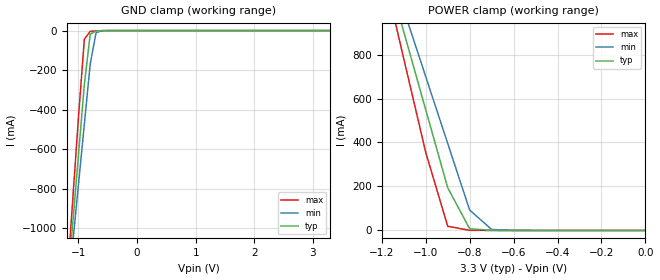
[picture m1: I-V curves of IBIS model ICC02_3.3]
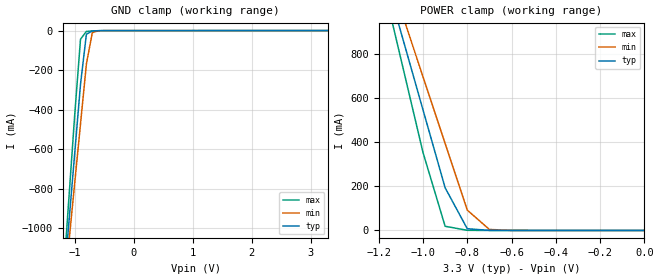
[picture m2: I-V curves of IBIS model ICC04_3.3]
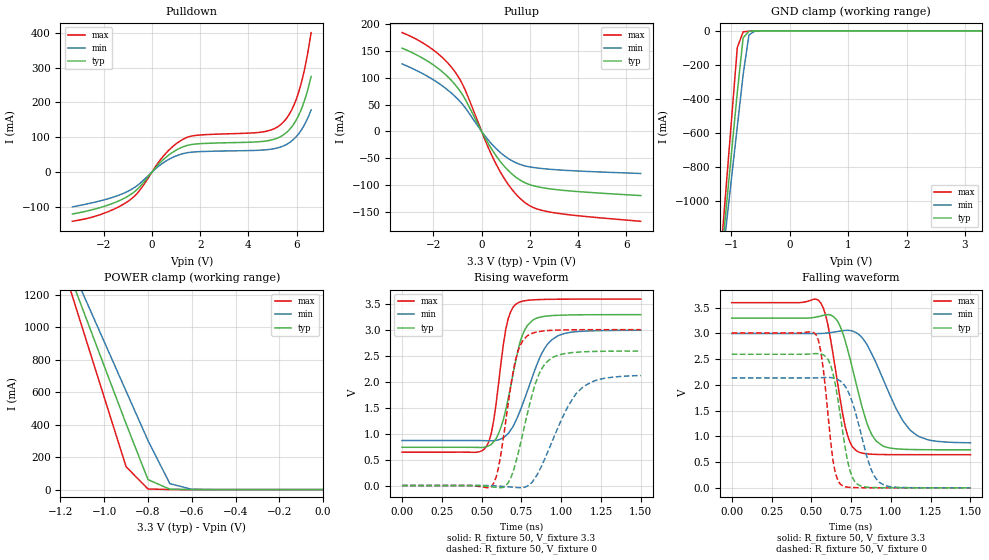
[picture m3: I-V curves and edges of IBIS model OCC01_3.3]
|   MPC9350   I B I S   M O D E L   |
|   F R E E S C A L E   S E M I C O N D U C T O R   |
[IBIS Ver]   3.2
[File name]   mpc9350.ibs
[File Rev]   1.0
[Date]   01-Apr-05 10:30:01 AM
[Source]   This file was generated from transistor-level
|   simulations
[Notes]   This file contains data for 3.3V and 2.5 V
|   applications.
[Disclaimer]   This information is for modeling purposes only,
|   and is not guaranteed.
[Copyright]   Copyright 2005, Freescale Semiconductor.,
|   All Rights Reserved.
|   MPC9350
|   --- 3.3V Application ---
|   C O M P O N E N T  D E S C R I P T I O N
[Component]   mpc9350_3.3v
[Manufacturer]   Freescale Semiconductor
[Package]
R_pkg   40m   40m   40m
L_pkg   0.5nH   0.5nH   0.5nH
C_pkg   0.23pF   0.23pF   0.23pF
[Pin] signal_name   model_name   R_pin   L_pin   C_pin
1   VCCA   POWER   40m   0.5nH   0.23pF
2   FBSEL   ICC04_3.3   40m   0.5nH   0.23pF
3   FSELA   ICC04_3.3   40m   0.5nH   0.23pF
4   FSELB   ICC04_3.3   40m   0.5nH   0.23pF
5   FSELC   ICC04_3.3   40m   0.5nH   0.23pF
6   FSELD   ICC04_3.3   40m   0.5nH   0.23pF
7   GND   GND   40m   0.5nH   0.23pF
|8   XTAL1   NA   40m   0.5nH   0.23pF
|9   XTAL2   NA   40m   0.5nH   0.23pF
10   OEB   ICC04_3.3   40m   0.5nH   0.23pF
11   VCCO   POWER   40m   0.5nH   0.23pF
12   QD4   OCC01_3.3   40m   0.5nH   0.23pF
13   GND   GND   40m   0.5nH   0.23pF
14   QD3   OCC01_3.3   40m   0.5nH   0.23pF
15   VCCO   POWER   40m   0.5nH   0.23pF
16   QD2   OCC01_3.3   40m   0.5nH   0.23pF
17   GND   GND   40m   0.5nH   0.23pF
18   QD1   OCC01_3.3   40m   0.5nH   0.23pF
19   VCCO   POWER   40m   0.5nH   0.23pF
20   QD0   OCC01_3.3   40m   0.5nH   0.23pF
21   GND   GND   40m   0.5nH   0.23pF
22   QC1   OCC01_3.3   40m   0.5nH   0.23pF
23   VCCO   POWER   40m   0.5nH   0.23pF
24   QC0   OCC01_3.3   40m   0.5nH   0.23pF
25   GND   GND   40m   0.5nH   0.23pF
26   QB   OCC01_3.3   40m   0.5nH   0.23pF
27   VCCO   POWER   40m   0.5nH   0.23pF
28   QA   OCC01_3.3   40m   0.5nH   0.23pF
29   GND   GND   40m   0.5nH   0.23pF
30   TCLK   ICC04_3.3   40m   0.5nH   0.23pF
31   PLL_EN   ICC02_3.3   40m   0.5nH   0.23pF
32   REF_SEL   ICC04_3.3   40m   0.5nH   0.23pF
|[Diff Pin] inv_pin vdiff   tdelay_typ tdelay_min tdelay_max
|8   9   0.0   0.0   0.0   0.0
|   MPC9350
|   --- 2.5V Application ----
|   C O M P O N E N T  D E S C R I P T I O N
[Component]   mpc9350_2.5v
[Manufacturer]   Freescale Semiconductor
[Package]
R_pkg   40m   40m   40m
L_pkg   0.5nH   0.5nH   0.5nH
C_pkg   0.23pF   0.23pF   0.23pF
[Pin] signal_name   model_name   R_pin   L_pin   C_pin
1   VCCA   POWER   40m   0.5nH   0.23pF
2   FBSEL   ICC04_2.5   40m   0.5nH   0.23pF
3   FSELA   ICC04_2.5   40m   0.5nH   0.23pF
4   FSELB   ICC04_2.5   40m   0.5nH   0.23pF
5   FSELC   ICC04_2.5   40m   0.5nH   0.23pF
6   FSELD   ICC04_2.5   40m   0.5nH   0.23pF
7   GND   GND   40m   0.5nH   0.23pF
|8   XTAL1   NA   40m   0.5nH   0.23pF
|9   XTAL2   NA   40m   0.5nH   0.23pF
10   OEB   ICC04_2.5   40m   0.5nH   0.23pF
11   VCCO   POWER   40m   0.5nH   0.23pF
12   QD4   OCC01_2.5   40m   0.5nH   0.23pF
13   GND   GND   40m   0.5nH   0.23pF
14   QD3   OCC01_2.5   40m   0.5nH   0.23pF
15   VCCO   POWER   40m   0.5nH   0.23pF
16   QD2   OCC01_2.5   40m   0.5nH   0.23pF
17   GND   GND   40m   0.5nH   0.23pF
18   QD1   OCC01_2.5   40m   0.5nH   0.23pF
19   VCCO   POWER   40m   0.5nH   0.23pF
20   QD0   OCC01_2.5   40m   0.5nH   0.23pF
21   GND   GND   40m   0.5nH   0.23pF
22   QC1   OCC01_2.5   40m   0.5nH   0.23pF
23   VCCO   POWER   40m   0.5nH   0.23pF
24   QC0   OCC01_2.5   40m   0.5nH   0.23pF
25   GND   GND   40m   0.5nH   0.23pF
26   QB   OCC01_2.5   40m   0.5nH   0.23pF
27   VCCO   POWER   40m   0.5nH   0.23pF
28   QA   OCC01_2.5   40m   0.5nH   0.23pF
29   GND   GND   40m   0.5nH   0.23pF
30   TCLK   ICC04_2.5   40m   0.5nH   0.23pF
31   PLL_EN   ICC02_2.5   40m   0.5nH   0.23pF
32   REF_SEL   ICC04_2.5   40m   0.5nH   0.23pF
| Models and submodels in the file (6): ICC02_3.3 (Input), ICC04_3.3 (Input), OCC01_3.3 (3-state), ICC02_2.5 (Input), ICC04_2.5 (Input), OCC01_2.5 (3-state)
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|[Diff Pin] inv_pin vdiff   tdelay_typ tdelay_min tdelay_max
|8   9   0.0   0.0   0.0   0.0
|   M O D E L  S T A T E M E N T
|   ICC02_3.3: LVCMOS INPUT MODEL WITH A 25K PULLUP RESISTOR
[Model]   ICC02_3.3
Model_type  Input
Vinh   =  2.0
Vinl   =  0.8
C_comp   4pF   4pF   4pF
[Temperature Range] 55   110   0
[Voltage Range]   3.3   3.0   3.6
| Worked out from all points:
|   GND clamp passes 1 mA (typ) near -0.64 V on its own axis
|   POWER clamp passes 1 mA (typ) near -0.71 V on its own axis
[GND Clamp]
-3.3V     -8.818A    -7.792A    -10.27A
-1.2V     -1.34A     -1.387A    -1.291A
-1.1V     -983.9mA   -1.082A    -863.3mA
-1V       -628.2mA   -777.7mA   -436mA
-900mV    -272.6mA   -473.3mA   -43.61mA
-800mV    -18.37mA   -169.1mA   -4.071mA
-700mV    -1.803mA   -10.53mA   -1.748mA
-600mV    -469.6uA   -844.1uA   -549.6uA
3.3V      198.3pA    131.6nA    29.07pA
[POWER Clamp]
-3.3V     8.713A     7.69A      10.16A
-1.2V     1.258A     1.306A     1.207A
-1.1V     903mA      1.003A     780.7mA
-1V       548.5mA    699.1mA    354.8mA
-900mV    194.1mA    395.6mA    19.11mA
-800mV    7.956mA    92.59mA    801.4uA
-700mV    419.3uA    4.687mA    153.6uA
-600mV    61.5uA     290.9uA    36.86uA
0V        198.3pA    812.2pA    35.68pA
|   ICC04_3.3: LVCMOS INPUT MODEL WITH A 25K PULLDOWN RESISTOR
[Model]   ICC04_3.3
Model_type  Input
Vinh   =  2.0
Vinl   =  0.8
C_comp   4pF   4pF   4pF
[Temperature Range] 55   110   0
[Voltage Range]   3.3   3.0   3.6
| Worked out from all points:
|   GND clamp passes 1 mA (typ) near -0.64 V on its own axis
|   POWER clamp passes 1 mA (typ) near -0.71 V on its own axis
[GND Clamp]
-3.3V     -8.818A    -7.792A    -10.27A
-1.2V     -1.34A     -1.387A    -1.291A
-1.1V     -983.9mA   -1.082A    -863.3mA
-1V       -628.2mA   -777.7mA   -436mA
-900mV    -272.7mA   -473.4mA   -43.64mA
-800mV    -18.4mA    -169.2mA   -4.102mA
-700mV    -1.832mA   -10.56mA   -1.775mA
-600mV    -494uA     -870uA     -572.7uA
3.3V      134.5uA    142.7uA    127.3uA
[POWER Clamp]
-3.3V     8.713A     7.69A      10.16A
-1.2V     1.258A     1.306A     1.207A
-1.1V     902.9mA    1.003A     780.7mA
-1V       548.4mA    699mA      354.7mA
-900mV    194.1mA    395.6mA    19.08mA
-800mV    7.923mA    92.56mA    770.6uA
-700mV    390.8uA    4.657mA    126.6uA
-600mV    37.06uA    265uA      13.73uA
0V        198.3pA    812.2pA    35.68pA
|   OCC01_3.3: LVCMOS OUTPUT MODEL
[Model]   OCC01_3.3
Model_type   3-state
Enable   Active-Low
Polarity   Non-Inverting
Vmeas   =   1.65
C_comp   3.5pF   3.5pF   3.5pF
[Temperature Range] 55   110   0
[Voltage Range]   3.3   3.0   3.6
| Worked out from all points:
|   slope of the pulldown table from 0 to 0.495 V, typ, clamps not added: 13.2 ohm
|   slope of the pullup table from 0 to 0.495 V, typ, clamps not added: 12.8 ohm
|   GND clamp passes 1 mA (typ) near -0.62 V on its own axis
|   POWER clamp passes 1 mA (typ) near -0.64 V on its own axis
|   falling waveform, R_fixture 50, V_fixture 3.3: 20-80 % time 131ps typ, 192ps min, 96.1ps max; typ from 3.3 V to 0.739 V
|   falling waveform, R_fixture 50, V_fixture 0: 20-80 % time 82.2ps typ, 116ps min, 62.6ps max; typ from 2.6 V to 0 V
|   rising waveform, R_fixture 50, V_fixture 3.3: 20-80 % time 109ps typ, 160ps min, 76.6ps max; typ from 0.739 V to 3.3 V
|   rising waveform, R_fixture 50, V_fixture 0: 20-80 % time 130ps typ, 193ps min, 90.6ps max; typ from 0 V to 2.6 V
[Pullup]
-3.3V     155.4mA    126mA      184.5mA
-2V       124mA      96.25mA    151.9mA
-1.5V     106.1mA    80.65mA    132.3mA
-1.1V     87.3mA     65.18mA    110.9mA
-700mV    61.49mA    45.32mA    79.14mA
200mV     -16.79mA   -11.93mA   -22.35mA
700mV     -51.76mA   -36.33mA   -69.54mA
1.2V      -77.19mA   -53.3mA    -105mA
1.8V      -95.88mA   -64.45mA   -133mA
2.3V      -103.2mA   -68.31mA   -144.8mA
3V        -108.2mA   -71.3mA    -151.8mA
6.6V      -119.8mA   -78.56mA   -167.9mA
[Pulldown]
-3.3V     -120.3mA   -99.81mA   -141.2mA
-2V       -98.75mA   -80mA      -118.5mA
-900mV    -65.04mA   -51.45mA   -79.15mA
-500mV    -41.5mA    -32.23mA   -51.45mA
600mV     43.7mA     32.62mA    55.87mA
1.4V      75.31mA    54.8mA     98.02mA
4.5V      87.58mA    62.98mA    114.5mA
5.3V      100.7mA    71.34mA    134.3mA
5.7V      121.9mA    84.58mA    166.6mA
6V        151.7mA    103mA      212.2mA
6.3V      200mA      132.8mA    286.3mA
6.6V      274.6mA    178.5mA    400.7mA
[GND Clamp]
-3.3V     -8.925A    -7.897A    -10.38A
-1.2V     -1.43A     -1.477A    -1.382A
-1.1V     -1.074A    -1.171A    -953.9mA
-1V       -717.3mA   -866.4mA   -525.7mA
-900mV    -361.1mA   -561.5mA   -98.15mA
-800mV    -41.01mA   -256.9mA   -6.004mA
-700mV    -2.888mA   -24.01mA   -2.342mA
-600mV    -641.5uA   -1.609mA   -734.7uA
3.3V      264.6pA    572.4nA    37.87pA
[POWER Clamp]
-3.3V     9.003A     7.964A     10.47A
-1.2V     1.476A     1.523A     1.427A
-1.1V     1.119A     1.217A     998mA
-1V       762.3mA    912.1mA    569.3mA
-900mV    406mA      607.2mA    141.1mA
-800mV    61.63mA    302.7mA    3.873mA
-700mV    2.356mA    36.76mA    461.2uA
-600mV    158.8uA    1.918mA    48.48uA
0V        264.6pA    1.092nA    46.62pA
[Falling Waveform]
R_fixture=50
V_fixture=3.3
V_fixture_min=3.0
V_fixture_max=3.6
0s        3.3V       3V         3.6V
545.5ps   3.329V     2.998V     3.646V
590.9ps   3.362V     3.007V     3.348V
666.7ps   3.232V     3.039V     2.008V
727.3ps   2.697V     3.062V     1.023V
787.9ps   1.951V     3.006V     710.6mV
848.5ps   1.266V     2.792V     661.1mV
909.1ps   906.4mV    2.412V     650mV
1.121ns   745.3mV    1.121V     644.6mV
1.5ns     739.1mV    875.3mV    644.4mV
[Falling Waveform]
R_fixture=50
V_fixture=0
V_fixture_min=0
V_fixture_max=0
0s        2.597V     2.136V     3.01V
530.3ps   2.609V     2.137V     2.977V
575.8ps   2.584V     2.143V     2.3V
621.2ps   2.389V     2.143V     913.1mV
651.5ps   1.997V     2.125V     282.1mV
697ps     1.099V     2.036V     38.48mV
772.7ps   124.2mV    1.52V      5.2mV
863.6ps   10.2mV     467.9mV    1.186mV
924.2ps   4.231mV    114.1mV    447.5uV
1.5ns     4.564uV    187.7uV    234.6nV
[Rising Waveform]
R_fixture=50
V_fixture=3.3
V_fixture_min=3.0
V_fixture_max=3.6
0s        739mV      869.8mV    644.4mV
530.3ps   750.3mV    865.8mV    755.8mV
575.8ps   844.5mV    866.2mV    1.254V
651.5ps   1.461V     959.3mV    3.015V
681.8ps   1.904V     1.069V     3.351V
727.3ps   2.594V     1.334V     3.526V
787.9ps   3.094V     1.828V     3.577V
878.8ps   3.26V      2.558V     3.593V
939.4ps   3.281V     2.81V      3.597V
1.5ns     3.3V       2.999V     3.6V
[Rising Waveform]
R_fixture=50
V_fixture=0
V_fixture_min=0
V_fixture_max=0
0s        2.688nV    14.94nV    362.8pV
560.6ps   -23.19mV   -1.829mV   -22.02mV
606.1ps   -40.45mV   -10.02mV   348.4mV
681.8ps   136.8mV    -27.54mV   1.895V
727.3ps   592.2mV    -40.33mV   2.582V
787.9ps   1.395V     -9.759mV   2.893V
848.5ps   2.058V     205.8mV    2.966V
909.1ps   2.385V     603.5mV    2.991V
1.136ns   2.583V     1.903V     3.009V
1.5ns     2.597V     2.125V     3.01V
[Ramp]
R_load=50
dV/dt_r   1.558E+0/1.297E-10   1.275E+0/1.933E-10   1.806E+0/9.057E-11
dV/dt_f   1.537E+0/1.311E-10   1.275E+0/1.913E-10   1.773E+0/9.552E-11
|[End   OCC01_3.3
